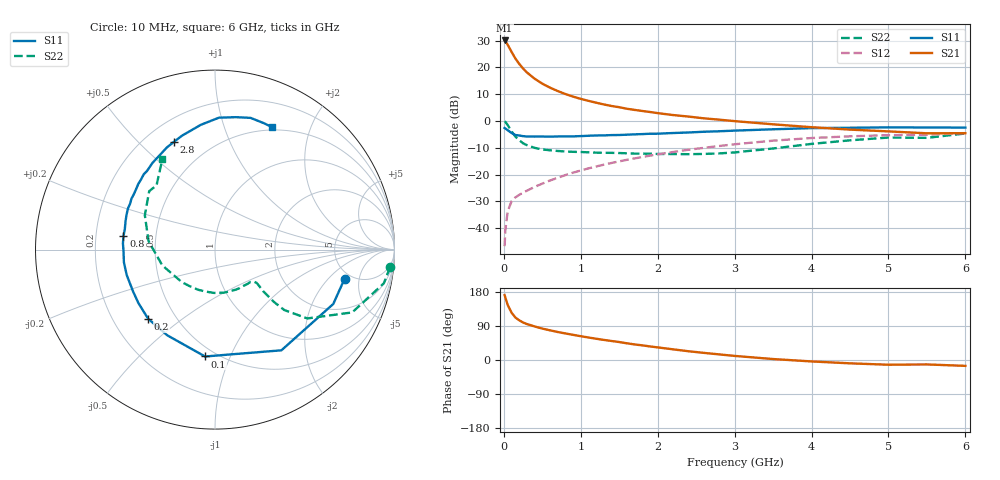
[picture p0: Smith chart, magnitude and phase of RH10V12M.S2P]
! SIEMENS Small Signal Semiconductors
! BFR106
! Si NPN RF Bipolar Junction Transistor in SOT23
! VCE = 10 V  IC = 12 mA
! Common Emitter S-Parameters:  August  1996
# GHz  S  MA  R  50
!  f  S11  S21  S12  S22
! GHz  MAG  ANG  MAG  ANG  MAG  ANG  MAG  ANG
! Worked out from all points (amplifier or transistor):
!   36 points, 10 MHz to 6 GHz, reference 50 ohm
!   highest |S21| = 30.1 dB at 10 MHz (marker M1)
!   |S21| within 3 dB of that: start of sweep to 76.64 MHz
!   unconditionally stable (mu >= 1): 475.1 MHz to 2.022 GHz; 5.457 GHz to 5.8 GHz
!   at 250 MHz: K = 0.75, MSG = 23.2 dB, |S12| = -26.8 dB
!   at 1.4 GHz: K = 1.08, MAG = 8.9 dB, |S12| = -15.7 dB
!   at 6 GHz: K = 1.00, MSG = 0.0 dB, |S12| = -4.5 dB
!   S11 on the Smith chart (normalised r, x): 10 MHz: 4.38, -3.13; 100 MHz: 0.44, -0.81; 200 MHz: 0.35, -0.38; 800 MHz: 0.32, +0.07; 2.8 GHz: 0.31, +0.64; 6 GHz: 0.47, +1.47
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0.01  0.7404 -12.6  31.85 171.3  0.0046 84.5  0.9808 -5.7
0.02  0.7252 -24.7  30.88 164.6  0.0093 79.5  0.9591 -11.3
0.05  0.6721 -56.6  26.51 145.1  0.0205 65.5  0.8407 -24.6
0.1  0.5981 -95.3  19.57 124.9  0.0317 53.8  0.6417 -36.7
0.15  0.5466 -119.1  14.64 112.1  0.0374 49.7  0.5122 -41.1
0.2  0.5359 -134.0  11.65 104.8  0.0418 49.9  0.4369 -41.6
0.25  0.5205 -145.0  9.525 98.9  0.0459 50.6  0.3832 -41.1
0.3  0.5127 -152.7  8.051 94.9  0.0499 52.8  0.3533 -40.8
0.4  0.5119 -163.9  6.163 88.5  0.0587 55.7  0.3152 -39.3
0.5  0.5125 -172.1  4.971 82.9  0.0677 58.5  0.2945 -38.6
0.6  0.5097 -178.8  4.186 78.3  0.0774 60.4  0.2837 -39.4
0.8  0.5155 171.6  3.182 70.1  0.0977 62.9  0.2689 -42.2
0.9  0.5153 167.1  2.847 66.4  0.1085 63.7  0.2655 -43.8
1.1  0.5295 158.6  2.375 59.4  0.1303 64.2  0.2599 -49.3
1.3  0.5378 151.5  2.035 53.0  0.153 63.9  0.2545 -55.0
1.6  0.5546 142.2  1.691 44.1  0.1884 62.5  0.2493 -65.5
2.2  0.5957 125.8  1.29 28.1  0.2637 57.1  0.2415 -91.1
2.8  0.6426 110.8  1.058 14.8  0.3413 49.3  0.2478 -124.9
3.5  0.6996 96.5  0.866 2.5  0.4292 38.7  0.3065 -163.3
4.5  0.7468 81.1  0.69 -8.8  0.5168 21.5  0.4352 153.9
5.5  0.7552 68.8  0.589 -11.7  0.5525 9.5  0.484 132.3
6  0.7528 64.9  0.592 -15.5  0.5928 1.5  0.584 120.1
